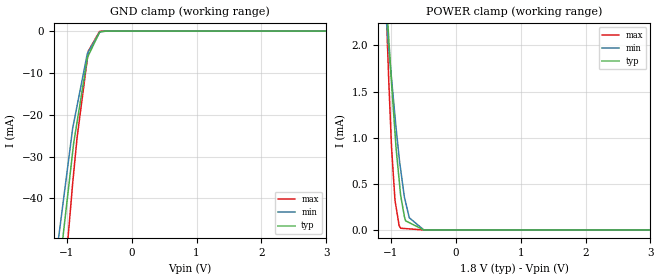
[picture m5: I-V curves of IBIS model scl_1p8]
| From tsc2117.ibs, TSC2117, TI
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|   scl_1p8 Model
[Model]   scl_1p8
Model_type   Input
Vinl = 0.54
Vinh = 1.26
|   typ   min   max
|   (nom PVT)   (fast PVT)   (slow PVT)
|C_comp from frequency sweep method (F=400KHz)
|Average
|C_comp   3.666e-12   3.640e-12   3.681e-12
|C_comp from LC tank measurement(L=1nH)
|Average
|Resonant Frequency(Hz)   4.620e+09   4.640e+09   4.617e+09
C_comp   1.188e-12   1.178e-12   1.189e-12
| Where nom  PVT is Nominal Process, 1.8V, 48C
|   Fast PVT is Strong Process,  1.98V, -40C
|   Slow PVT is Weak Process,   1.62V, 108C
[Model Spec]
|Subparameter   typ   min   max
Vinh   1.26   1.134   1.386
Vinl   0.54   0.486   0.594
[Voltage Range]   1.8   1.62   1.98
|Ambient Temperature   25   85   -40
|Junction Temperature
[Temperature Range]   48   108   -40
[Power Clamp Reference]   1.8   1.62   1.98
[GND Clamp Reference]   0   0   0
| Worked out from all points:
|   GND clamp passes 1 mA (typ) near -0.52 V on its own axis
|   POWER clamp passes 1 mA (typ) near -0.93 V on its own axis
[GND Clamp]
|   Voltage   I(typ)   I(min)   I(max)
-1.8V     -240.5mA   -130.8mA   -381.7mA
-1.135V   -59.46mA   -50.42mA   -77.52mA
-910.4mV  -29.03mA   -23.35mA   -36.59mA
-892.8mV  -26.66mA   -21.92mA   -33.72mA
-841.5mV  -21.74mA   -17.87mA   -25.51mA
-686.9mV  -6.885mA   -5.643mA   -7.097mA
-680.4mV  -6.263mA   -5.29mA    -6.326mA
-667.3mV  -5.837mA   -4.938mA   -4.761mA
-495mV    -260.5uA   -323.8uA   -73.08uA
-307.8mV  -1.423uA   -3.756uA   -100.3nA
3.6V      0A         0A         0A
[POWER Clamp]
|   Voltage   I(typ)   I(min)   I(max)
-1.8V     11.89mA    8.634mA    19.35mA
-1.085V   2.686mA    2.385mA    2.616mA
-1.035V   2.081mA    1.973mA    1.633mA
-990mV    1.577mA    1.628mA    881.4uA
-938.5mV  1.059mA    1.234mA    323.2uA
-919.8mV  874.1uA    1.094mA    242.3uA
-875.2mV  549.7uA    793.1uA    49.36uA
-851.4mV  377uA      658uA      18.85uA
-774mV    98.6uA     299.2uA    14.76uA
-717.7mV  78.69uA    132uA      11.78uA
-494.1mV  14.85nA    598.8nA    0A
3.6V      0A         0A         0A
